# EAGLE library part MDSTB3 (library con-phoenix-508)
PHOENIX
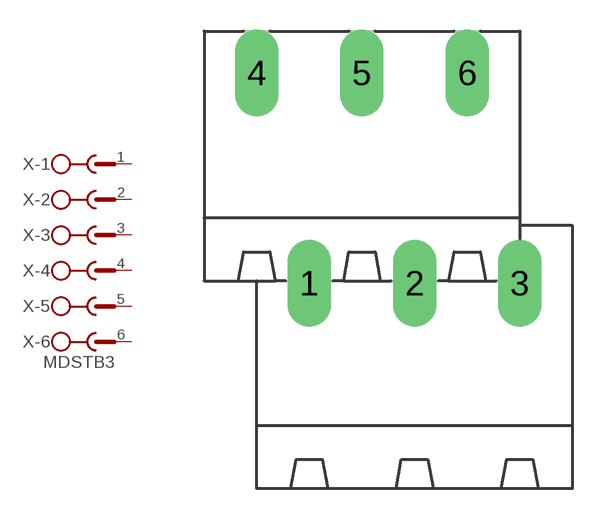
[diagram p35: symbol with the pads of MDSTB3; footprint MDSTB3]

Designator prefix X; gates -1=SK -2=SK -3=SK -4=SK -5=SK -6=SKV

## MDSTB3 (OC_FARNELL: unknown; OC_NEWARK: unknown)  [MDSTB3]
1  -1:1  pas
2  -2:1  pas
3  -3:1  pas
4  -4:1  pas
5  -5:1  pas
6  -6:1  pas

## Footprint MDSTB3 (pad centres in mm)
PHOENIX
drill 1.397 long: 1 -3.81,-5.08; 2 1.27,-5.08; 3 6.35,-5.08; 4 -6.35,5.08; 5 -1.27,5.08; 6 3.81,5.08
